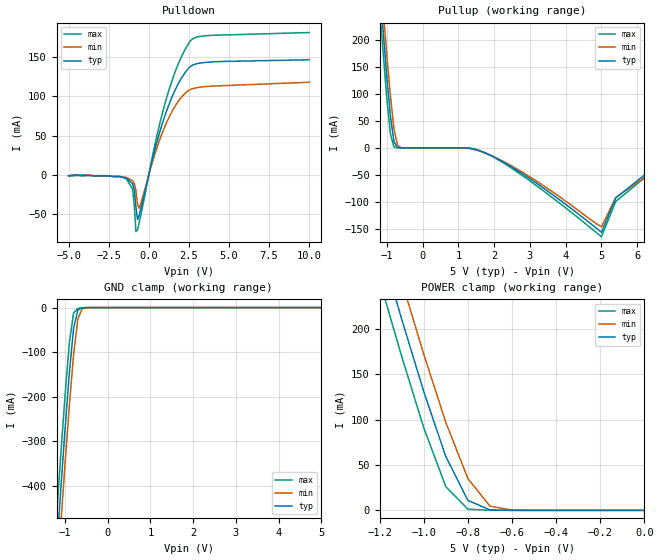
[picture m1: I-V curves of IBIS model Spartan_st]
|   * spartan_st.ibs * IBIS 1.1 Model for Spartan
[IBIS Ver]	1.1
[Comment char]	|_char
[File name]	spartan_st.ibs
[Date]		Thu Jan 22 17:48:24 1998
[File Rev]	1.0
[Source] s2ibis Version 1.0 SPICE to IBIS converter
   s05-1e.lib, s05-1ediode.mod
[Notes]   Spartan 5V process
[Disclaimer]
The data in this model is derived from SPICE simulations using modeling
information extracted from the target process.  While a great deal of
care has been taken to provide information that is accurate, this model
is considered preliminary as it has not been verified by actual silicon
measurement.  Treat the data in this model as preliminary until actual
silicon verification is performed.
| Spartan - Slow, TTL
|   COMPONENT: Spartan
[Component]	Spartan
[Manufacturer]	Xilinx
[Package]
| Note: approximate package data for PQ's
|   typ   min   max
R_pkg   60m   40m   80m
L_pkg   13nH   10nH   16nH
C_pkg   1.4pF   0.7pF   2pF
[Pin] signal_name model_name R_pin L_pin C_pin
all   iob   Spartan_st
2 GND GND
3 VDD POWER
| Models and submodels in the file (1): Spartan_st (I/O)
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|   MODEL Spartan_st
[Model]		Spartan_st
Model_type	I/O
Polarity	Non-Inverting
Enable		Active-Low
Vinh  = 2.0V
Vinl  = 0.8V
C_comp   7.0p   5.0p   9.0p
[Voltage range]   5.000   4.500   5.500
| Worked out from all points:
|   slope of the pulldown table from 0 to 0.75 V, typ, clamps not added: 12.8 ohm
|   GND clamp passes 1 mA (typ) near -0.61 V on its own axis
|   POWER clamp passes 1 mA (typ) near -0.70 V on its own axis
[Pulldown]
|  Voltage   I(typ)   I(min)   I(max)
-5V       -1mA       -1mA       -1mA
-1.4V     -3.9mA     -3.1mA     -4.7mA
-1V       -11.3mA    -7.5mA     -18.3mA
-900mV    -19.4mA    -11.3mA    -39.37mA
-800mV    -40.4mA    -19.7mA    -71.92mA
-700mV    -56.79mA   -37mA      -69.71mA
-600mV    -51.51mA   -42.23mA   -60.92mA
400mV     33.53mA    27.75mA    40.02mA
1.1V      80.62mA    65.99mA    97.02mA
1.9V      118mA      95.03mA    143.8mA
2.6V      137.7mA    108.5mA    170.3mA
10V       146.2mA    117.6mA    180.7mA
[GND_clamp]
|  Voltage   I(typ)   I(min)   I(max)
-5V       -6.234A    -6.302A    -6.168A
-1.2V     -547.5mA   -626.3mA   -469.9mA
-1.1V     -407.8mA   -486.4mA   -330.4mA
-1V       -272.7mA   -350.3mA   -197.1mA
-900mV    -147.2mA   -220.8mA   -79.43mA
-800mV    -46.44mA   -105.5mA   -11.87mA
-700mV    -5.189mA   -25.6mA    -1.885mA
-600mV    -708.8uA   -2.512mA   -491.3uA
-500mV    -139.3uA   -303.7uA   -65.15uA
5V        150.7pA    16.26uA    111.2pA
[Pullup]
|  Voltage   I(typ)   I(min)   I(max)
-5V       3.726A     3.76A      3.696A
-1.4V     466.1mA    507.5mA    425.7mA
-1V       130.6mA    171.7mA    90.75mA
-900mV    59.08mA    96.7mA     26.03mA
-800mV    11mA       35.01mA    1.281mA
-700mV    518.3uA    4.623mA    24.8uA
-600mV    18.94uA    279.5uA    472.7nA
1.7V      -8.125mA   -8.403mA   -7.823mA
3V        -57.23mA   -53.76mA   -61.21mA
5V        -156.4mA   -146.5mA   -164.8mA
5.4V      -92.9mA    -91.72mA   -99.32mA
10V       150.9mA    118mA      151.8mA
[POWER_clamp]
|  Voltage   I(typ)   I(min)   I(max)
-5V       3.726A     3.76A      3.696A
-1.2V     293.8mA    335.7mA    252.7mA
-1.1V     210.3mA    252.2mA    169.3mA
-1V       130.6mA    171.7mA    90.75mA
-900mV    59.07mA    96.7mA     26.03mA
-800mV    10.99mA    35.01mA    1.277mA
-700mV    516uA      4.619mA    24.5uA
-600mV    18.72uA    277.8uA    467.8nA
0V        150.7pA    780.8pA    133.6pA
[Ramp]
|  variable   typ   min   max
dV/dt_r   1.32/3.70n   1.05/4.22n   1.59/3.12n
dV/dt_f   2.33/2.30n   1.95/3.02n   2.68/1.77n
